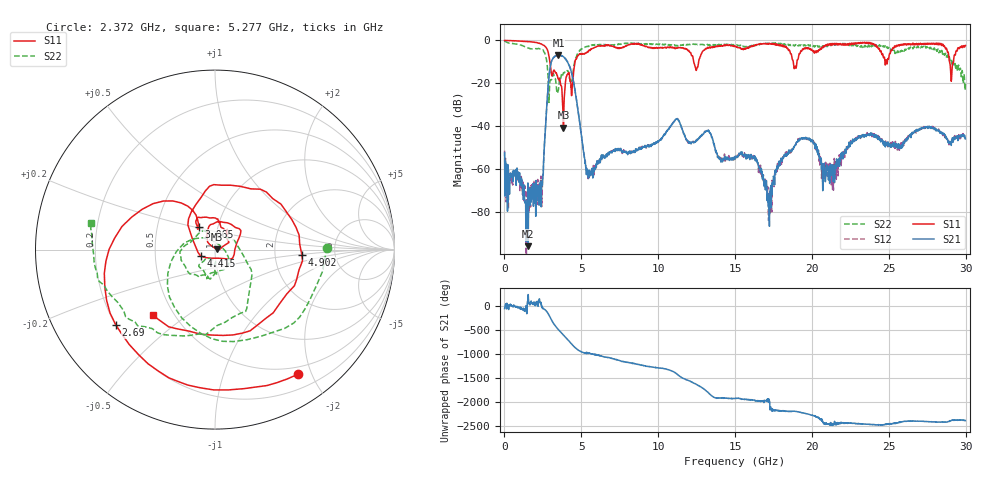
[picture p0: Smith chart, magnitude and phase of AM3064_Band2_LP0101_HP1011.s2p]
# Hz S DB R 50.0
!freq dBS11 angS11 dBS21 angS21 dBS12 angS12 dBS22 angS22
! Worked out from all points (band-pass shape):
!   1600 points, 10 MHz to 29.98 GHz, reference 50 ohm
!   highest |S21| = -6.76 dB at 3.515 GHz (marker M1); lowest = -95.8 dB at 1.547 GHz (marker M2)
!   |S21| within 3 dB of the highest: 3.059 GHz to 4.073 GHz (1.014 GHz wide, 28.4 % of centre)
!   lowest |S11| = -40.6 dB at 3.834 GHz (marker M3), VSWR 1.02, Z = 50.9 + j0.276 ohm
!   |S11| at or under -10 dB: 2.955 GHz to 4.593 GHz (1.638 GHz wide, 43.4 % of centre); 12.31 GHz to 12.63 GHz (321.2 MHz wide, 2.58 % of centre); 28.95 GHz to 29.2 GHz (255.4 MHz wide, 0.878 % of centre)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
!   |S22| runs from -28.9 to -0.3 dB; largest |S21 - S12| = 0.011
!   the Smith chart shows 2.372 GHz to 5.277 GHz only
!   S11 on the Smith chart (normalised r, x): 2.372 GHz: 0.39, -1.80; 2.69 GHz: 0.20, -0.32; 3.065 GHz: 0.81, +0.21; 4.415 GHz: 0.85, -0.06; 4.902 GHz: 2.86, -0.21; 5.277 GHz: 0.38, -0.37
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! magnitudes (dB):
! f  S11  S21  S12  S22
! 10 MHz  -0.1  -52.4  -51.4  -0.3
! 1.547 GHz  -0.6  -95.8  -71.8  -3.6
! 2.372 GHz  -1.6  -65.5  -63.2  -4.1
! 2.69 GHz  -3.2  -37.7  -37.7  -7.5
! 3.065 GHz  -16.1  -9.6  -9.6  -18.3
! 3.515 GHz  -18.0  -6.8  -6.8  -22.7
! 3.834 GHz  -40.6  -7.6  -7.6  -15.1
! 4.415 GHz  -21.1  -16.5  -16.5  -18.0
! 4.902 GHz  -6.3  -38.8  -38.7  -4.7
! 5.015 GHz  -6.6  -44.8  -44.5  -4.2
! 5.277 GHz  -5.9  -58.1  -57.6  -3.1
! 10 GHz  -3.5  -47.3  -46.9  -1.9
! 11.22 GHz  -3.7  -36.7  -36.5  -2.3
! 15 GHz  -2.7  -54.8  -55.3  -1.9
! 16.3 GHz  -2.2  -55.1  -54.4  -2.2
! 17.24 GHz  -1.4  -86.6  -77.5  -1.4
! 18.19 GHz  -2.4  -53.7  -53.2  -1.9
! 19.99 GHz  -4.4  -46.3  -46.9  -2.2
! 21.25 GHz  -1.5  -62.2  -67.2  -2.4
! 23.16 GHz  -1.0  -44.7  -45.7  -3.2
! 25 GHz  -8.4  -48.2  -47.9  -3.3
! 29.98 GHz  -2.4  -45.9  -45.9  -20.2
